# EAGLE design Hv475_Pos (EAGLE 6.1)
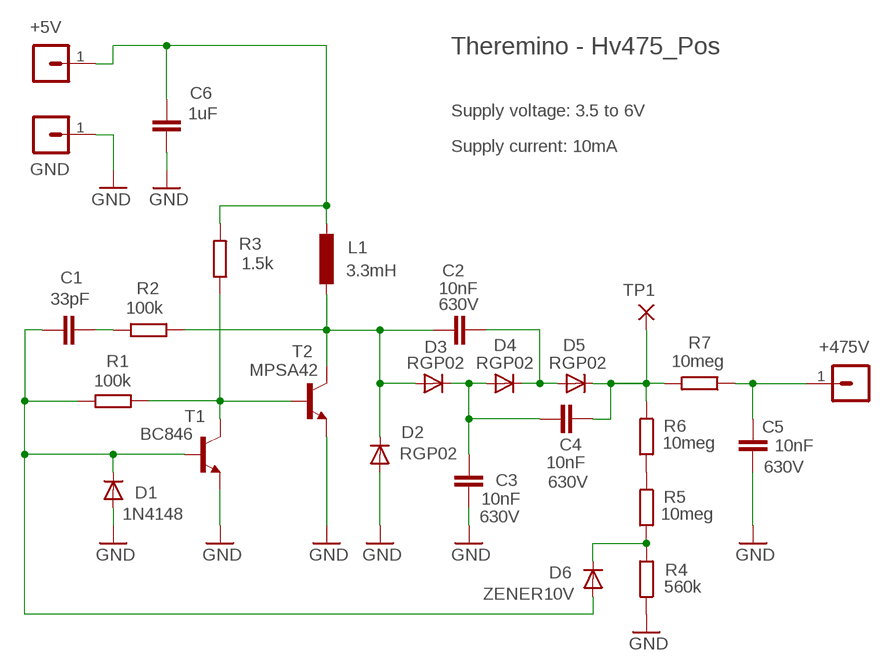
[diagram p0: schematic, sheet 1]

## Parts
+5V  MA01-1  [MA01-1]
+475V  MA01-1  [MA01-1]
C1  33pF  C-EU025-024X044  [C025-024X044]
C2  10nF  C-EU050-024X044  [C050-024X044]
C3  10nF  C-EU050-024X044  [C050-024X044]
C4  10nF  C-EU050-024X044  [C050-024X044]
C5  10nF  C-EU050-024X044  [C050-024X044]
C6  1uF  C-EUC0805  [C0805]
D1  1N4148  DIODE-DO34-7  [DO34-7]
D2  RGP02  DIODE-DO34-7  [DO34-7]
D3  RGP02  DIODE-DO34-7  [DO34-7]
D4  RGP02  DIODE-DO34-7  [DO34-7]
D5  RGP02  DIODE-DO34-7  [DO34-7]
D6  ZENER10V  DIODE-DO34-7  [DO34-7]
GND  MA01-1  [MA01-1]
L1  3.3mH  INDUCTORL_VERT_508  [L_VERT_508]
R1  100k  R-EU_0204/7  [0204/7]
R2  100k  R-EU_0204/7  [0204/7]
R3  1.5k  R-EU_0204/7  [0204/7]
R4  560k  R-EU_0204/7  [0204/7]
R5  10meg  R-EU_0204/7  [0204/7]
R6  10meg  R-EU_0204/7  [0204/7]
R7  10meg  R-EU_0204/7  [0204/7]
T1  BC846  -NPN-TO92-CBE  [TO92-CBE]
T2  MPSA42  -NPN-TO92-EBC  [TO92-EBC]
TP1  TEST  WIREPAD1,6/0,8  [1,6/0,8]

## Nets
+5V: +5V.1 C6.1 L1.+ R3.2
GND: C3.1 C5.1 C6.2 D1.A D2.A GND.1 R4.1 T1.E T2.E
N$1: D6.C R4.2 R5.2
N$2: C1.2 R2.2
N$3: R5.1 R6.2
N$4: C1.1 D1.C D6.A R1.2 T1.B
N$5: C4.2 D5.C R6.1 R7.2 TP1.1(P)
N$6: C2.1 D2.C D3.A L1.- R2.1 T2.C
N$11: C3.2 C4.1 D3.C D4.A
N$15: +475V.1 C5.2 R7.1
N$17: C2.2 D4.C D5.A
N$26: R1.1 R3.1 T1.C T2.B

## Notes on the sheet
- Theremino - Hv475_Pos
- Supply voltage: 3.5 to 6V
- Supply current: 10mA

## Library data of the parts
+5V +475V GND = 03-con-lstb-M:MA01-1: PIN HEADER
C1 C6 = 00-LIVIO:C-EU: CAPACITOR, European symbol
C2-C5 = 00-LIVIO:C-EU: CAPACITOR, European symbol; VOLTAGE: 630V
D1-D5 = 00-LIVIO:DIODE-: DIODE
D6 = 00-LIVIO:DIODE-: DIODE; VZ: 10V
L1 = 00-LIVIO:INDUCTOR
R1-R7 = 00-LIVIO:R-EU_: RESISTOR, European symbol
T1 T2 = 00-LIVIO:*-NPN-: NPN Transistror
TP1 = 00-LIVIO:WIREPAD: Wire PAD connect wire on PCB

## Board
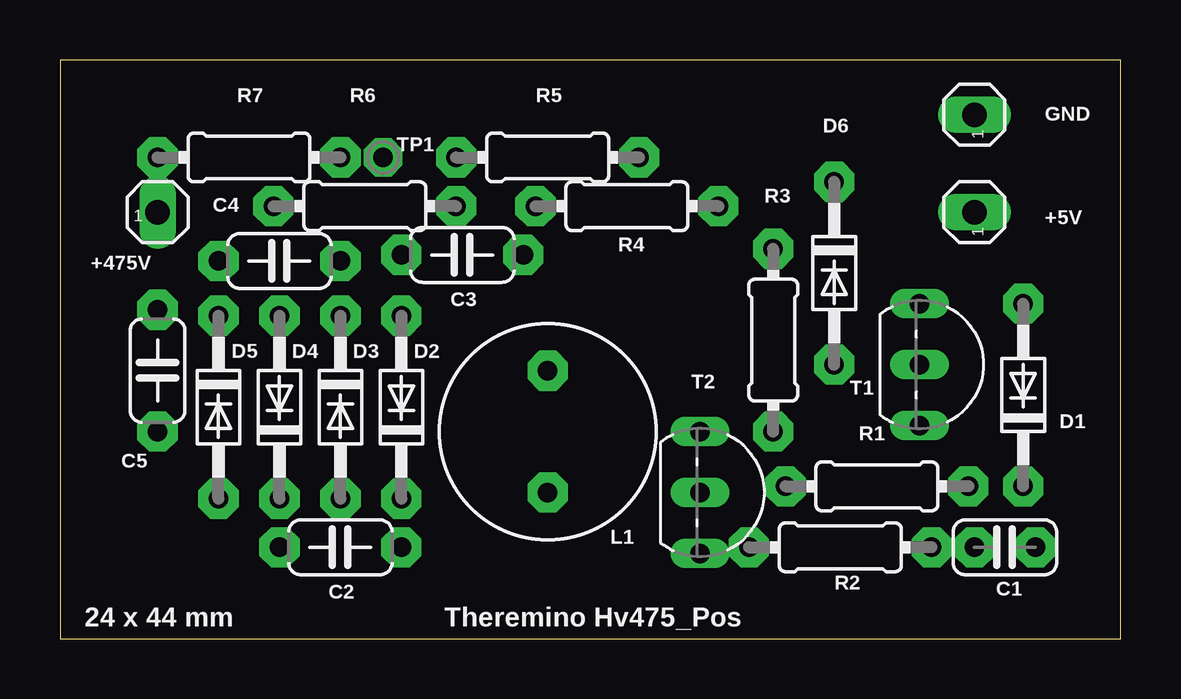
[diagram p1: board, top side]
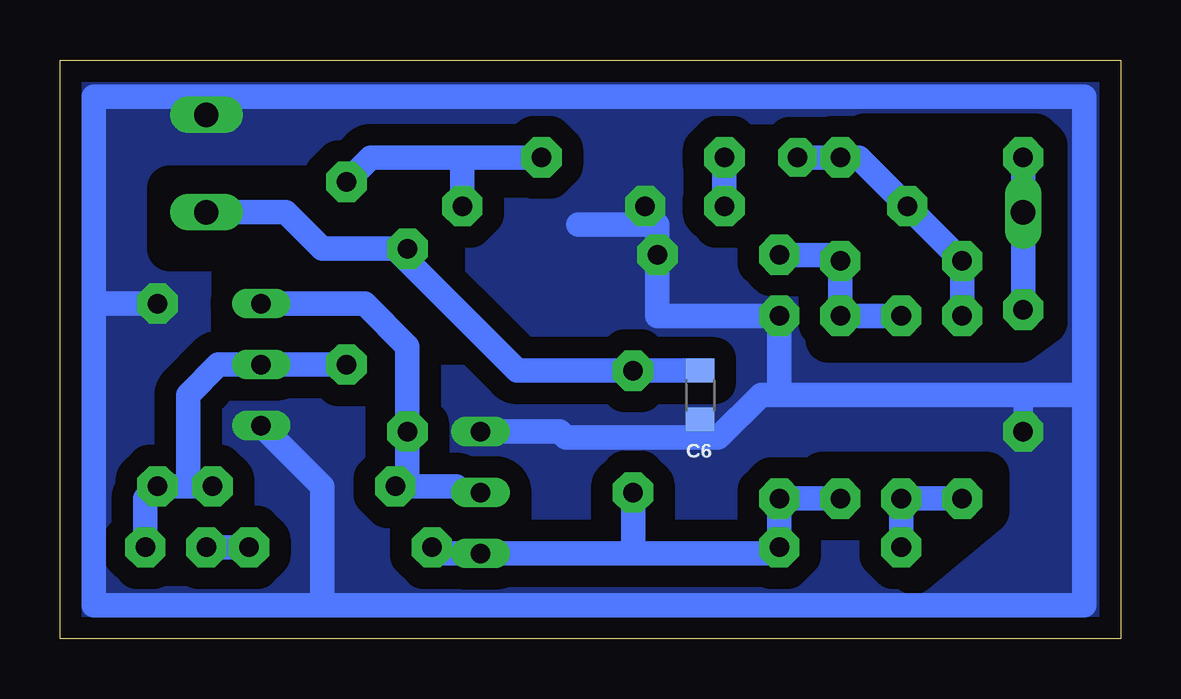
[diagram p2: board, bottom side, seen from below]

Size 44.2 x 24.13 mm. Coordinates in mm from the lower left corner, seen from the top.
Outline: 0,0 44.2,0 44.2,24.13 0,24.13 0,0
Copper layers (1*16): Top 0.035mm / dielectric 1.5mm / Bottom 0.035mm
Design rules: minimum track width 10mil, minimum drill 27mil, track to track 27mil, track to pad 27mil, pad to pad 27mil, via to via 27mil, smd to smd 27mil, copper to edge 27mil, drill to drill 8mil, minimum pad ring 5mil, minimum via ring 8mil, stop-mask expansion 4mil, vias tented up to drill 0mil, thermal gap 41mil
bRestrict: 11 lines

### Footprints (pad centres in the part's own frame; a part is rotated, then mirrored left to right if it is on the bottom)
MA01-1 = drill 1.016 long: 1 0,0
C025-024X044 = drill 0.813 pad 1.676 octagon: 1 -1.27,0; 2 1.27,0
C050-024X044 = drill 0.813 pad 1.676 octagon: 1 -2.54,0; 2 2.54,0
C0805 = smd 1 x 1.2: 1 -1.016,0; 2 1.016,0
DO34-7 = drill 0.813 pad 1.676 octagon: A 3.81,0; C -3.81,0
L_VERT_508 = drill 0.813 pad 1.676 octagon: + -2.54,0; - 2.54,0
0204/7 = drill 0.813 pad 1.676 octagon: 1 -3.81,0; 2 3.81,0
TO92-CBE = drill 0.813 long: B 0,0; C -2.54,0; E 2.54,0
TO92-EBC = drill 0.813 long: B 0,0; C 2.54,0; E -2.54,0
1,6/0,8 = drill 0.813 pad 1.6 octagon: 1 0,0

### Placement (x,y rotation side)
+5V  38.1,17.78 90 top
+475V  4.06,17.78 0 top
C1  39.37,3.81 180 top
C2  11.68,3.81 180 top
C3  16.76,16 180 top
C4  9.14,15.75 180 top
C5  4.06,11.18 90 top
C6  17.53,10.16 270 bottom
D1  40.13,10.16 90 top
D2  14.22,9.65 90 top
D3  11.68,9.65 270 top
D4  9.14,9.65 90 top
D5  6.6,9.65 270 top
D6  32.26,15.24 270 top
GND  38.1,21.84 90 top
L1  20.32,8.64 270 top
R1  34.04,6.35 0 top
R2  32.51,3.81 0 top
R3  29.72,12.45 90 top
R4  23.62,18.03 0 top
R5  20.32,20.07 0 top
R6  12.7,18.03 0 top
R7  7.87,20.07 0 top
T1  35.81,11.43 270 top
T2  26.67,6.1 270 top
TP1  13.46,20.07 180 top

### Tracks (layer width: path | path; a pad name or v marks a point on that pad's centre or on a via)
+5V
  Bottom 1.016: C6.1 L1.+ 25.15,11.18 30.23,16.26 R3.2 33.27,16.26 34.8,17.78 +5V.1
GND
  Bottom 0.813: C5.1 4.06,10.16
  Bottom 1.016: 17.53,8.38 23.11,8.38 23.37,8.64 T2.E | 14.22,10.16 4.06,10.16 1.52,10.16 | 33.27,1.4 1.52,1.4 1.52,10.16 | 33.27,1.4 42.8,1.4 42.8,13.97 | 42.8,13.97 42.8,22.61 1.52,22.61 1.52,10.16 | T1.E 33.27,6.35 33.27,1.4 | 22.61,17.27 19.3,17.27 C3.1 19.3,13.46 D2.A 14.22,10.16 | D1.A 42.8,13.97 | C6.2 17.53,8.38 | 17.53,8.38 16.76,8.38 14.99,10.16 14.22,10.16
  pour Bottom (isolate 0.9, rank 6, no thermals): -1,-1 45.2,-1 45.2,25.13 -1,25.13
N$1
  Bottom 1.016: R5.2 27.43,20.07 | 27.43,20.07 31.24,20.07 D6.C | R4.2 27.43,20.07
N$2
  Bottom 1.016: R2.2 C1.2
N$3
  Bottom 1.016: R6.2 R5.1
N$4
  Bottom 1.016: C1.1 40.64,5.84 D1.C 38.86,6.35 | 38.86,6.35 R1.2 | 38.86,6.35 38.86,10.16 37.59,11.43 T1.B D6.A
N$5
  Bottom 1.016: TP1.1 R7.2 10.92,20.07 R6.1 C4.2 D5.C
N$6
  Bottom 1.016: 20.32,3.56 14.22,3.56 C2.1 D2.C D3.A | 20.32,3.56 L1.- | 20.32,3.56 T2.C 28.7,3.56 R2.1
N$11
  Bottom 1.016: C3.2 11.68,16 C4.1 D3.C D4.A
N$15
  Bottom 1.016: R7.1 +475V.1 C5.2
N$17
  Bottom 1.016: C2.2 D4.C D5.A
N$26
  Bottom 1.016: T2.B 27.43,6.1 27.69,6.35 29.72,6.35 | 29.72,6.35 R1.1 29.72,6.35 | T1.C 31.5,13.97 29.72,12.19 R3.1 29.72,6.35

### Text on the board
tNames: 24 x 44 mm | Theremino Hv475_Pos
